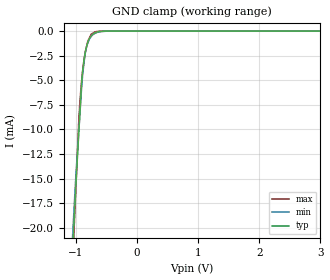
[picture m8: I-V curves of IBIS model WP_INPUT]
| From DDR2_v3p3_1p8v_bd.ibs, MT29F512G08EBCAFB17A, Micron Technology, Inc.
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| MODEL WP_INPUT (WP Input Model)
[Model]   WP_INPUT
Model_type   Input
Vinl = 360.000mV
Vinh = 1.440V
|   typ   min   max
|C_comp   2.250pF   2.150pF   2.350pF
C_comp_power_clamp   1.1250pF   1.0750pF   1.1750pF
C_comp_gnd_clamp   1.1250pF   1.0750pF   1.1750pF
[Model Spec]
| Input threshold voltage corners
Vinl   0.3600V   0.3400V   0.3900V
Vinh   1.4400V   1.3600V   1.5600V
| Dynamic Overshoot Parameters from ONFI4 Specification
D_overshoot_ampl_h   1.00   NA   NA
D_overshoot_ampl_l   1.00   NA   NA
D_overshoot_area_h   3.0n   NA   NA
D_overshoot_area_l   3.0n   NA   NA
[Voltage Range]   1.8000V   1.7000V   1.9500V
| Junction Temperature (Ambient temp is 35C typ, 70C min, 0C max)
[Temperature Range]   50.0   85.0   0.0
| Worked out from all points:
|   GND clamp passes 1 mA (typ) near -0.80 V on its own axis
[GND Clamp]
|   Voltage   I(typ)   I(min)   I(max)
-1.8V     -137.9mA   -123.9mA   -159.5mA
-1.06V    -23.14mA   -21.24mA   -24.59mA
-1.05V    -21.83mA   -20.09mA   -23.01mA
-1.04V    -20.52mA   -18.94mA   -21.45mA
-1.03V    -19.21mA   -17.79mA   -19.91mA
-950mV    -9.795mA   -9.676mA   -8.492mA
-910mV    -5.326mA   -5.887mA   -5.166mA
-890mV    -3.979mA   -4.329mA   -3.934mA
-840mV    -1.849mA   -1.953mA   -1.905mA
-740mV    -398.4uA   -466.2uA   -265.1uA
-490mV    -3.609uA   -5.756uA   -433.7nA
3.6V      0A         0A         0A
[POWER Clamp]
|   Voltage   I(typ)   I(min)   I(max)
-1.8V     0A         0A         0A
0V        0A         0A         0A
3.6V      0A         0A         0A
